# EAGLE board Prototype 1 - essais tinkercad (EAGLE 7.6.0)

Size 73.58 x 63.39 mm. Coordinates in mm from the lower left corner, seen from the top.
Outline: 0,0 56.82,0 56.82,53.33 0,53.33 0,0
Copper layers (1*16): Top 0.035mm / dielectric 1.5mm / Bottom 0.035mm
Design rules "default": minimum track width 10mil, minimum drill 24mil, track to track 8mil, track to pad 8mil, pad to pad 8mil, via to via 8mil, smd to smd 8mil, copper to edge 40mil, drill to drill 8mil, minimum pad ring 10mil, minimum via ring 8mil, stop-mask expansion 4mil, vias tented up to drill 0mil, thermal gap 10mil

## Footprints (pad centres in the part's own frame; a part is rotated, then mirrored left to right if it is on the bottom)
PIEZO-22MM = drill 1 pad 2.54: P$1 -5,0; P$2 5,0
1X3P-2.54-2.54-11.6-3.0-BLACK-MALE = drill 0.889 pad 1.651 square: 1 0,2.54 | drill 0.889 pad 1.651: 2 0,0; 3 0,-2.54
0207/10 = drill 0.813 octagon: 1 -5.08,0; 2 5.08,0
ARDUINO_UNO = drill 1.016 pad 1.88: 0 63.5,50.8; 1 60.96,50.8; 2 58.42,50.8; 3 55.88,50.8; 3.3V 35.56,2.54; 4 53.34,50.8; 5 50.8,50.8; 5V 38.1,2.54; 6 48.26,50.8; 7 45.72,50.8; 8 41.656,50.8; 9 39.116,50.8; 10 36.576,50.8; 11 34.036,50.8; 12 31.496,50.8; 13 28.956,50.8; A0 50.8,2.54; A1 53.34,2.54; A2 55.88,2.54; A3 58.42,2.54; A4 60.96,2.54; A5 63.5,2.54; AREF 23.876,50.8; GND 26.416,50.8; GND. 43.18,2.54; GND.. 40.64,2.54; I/OREF 30.48,2.54; N/C 27.94,2.54; RESET 33.02,2.54; SCL 18.796,50.8; SDA 21.336,50.8; VIN 45.72,2.54 | hole 3.2: 66.04,7.62; 66.04,35.56; 15.24,50.8; 13.97,2.54
1X16P-2.54-2.54-11.6-3.0-BLACK-MALE = drill 0.889 pad 1.651 square: 1 0,19.05 | drill 0.889 pad 1.651: 2 0,16.51; 3 0,13.97; 4 0,11.43; 5 0,8.89; 6 0,6.35; 7 0,3.81; 8 0,1.27; 9 0,-1.27; 10 0,-3.81; 11 0,-6.35; 12 0,-8.89; 13 0,-11.43; 14 0,-13.97; 15 0,-16.51; 16 0,-19.05

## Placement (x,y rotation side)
PIEZO2  [PIEZO-22MM]  not placed on the board
PIR1  [1X3P-2.54-2.54-11.6-3.0-BLACK-MALE]  5,48.18 0 top
PIR2  [1X3P-2.54-2.54-11.6-3.0-BLACK-MALE]  5,35.48 0 top
R3  220‎Ω  [0207/10]  5,60.88 0 top
U1  [ARDUINO_UNO]  5,10.08 0 top
U2  [1X16P-2.54-2.54-11.6-3.0-BLACK-MALE]  5,22.78 0 top

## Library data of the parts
PIEZO2 PIR1 PIR2 R3 U1 U2 = AUTODESK_CIRCUITS_BREADBOARD

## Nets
N$1: R3.1 U2.15
N$2: U1.2 U2.14
N$3: U1.3 U2.13
N$4: U1.4 U2.12
N$5: U1.5 U2.11
N$6: U1.7 U2.4
N$7: U1.6 U2.6
N$8: U1.A0 U2.3
N$9: PIEZO2.P$2 PIR1.1 PIR2.1 U1.GND U2.1 U2.5 U2.16
N$10: PIEZO2.P$1 U1.13
N$11: PIR1.3 U1.10
N$12: PIR2.3 U1.9
N$13: PIR2.2 U1.8
N$14: PIR1.2 U1.11
N$15: R3.2 U1.5V U2.2

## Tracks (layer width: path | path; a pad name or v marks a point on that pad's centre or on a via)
N$1  (1 unrouted)
N$2  (1 unrouted)
N$3  (1 unrouted)
N$4  (1 unrouted)
N$5  (1 unrouted)
N$6  (1 unrouted)
N$7  (1 unrouted)
N$8  (1 unrouted)
N$9  (6 unrouted)
N$10  (1 unrouted)
N$11  (1 unrouted)
N$12  (1 unrouted)
N$13  (1 unrouted)
N$14  (1 unrouted)
N$15  (2 unrouted)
